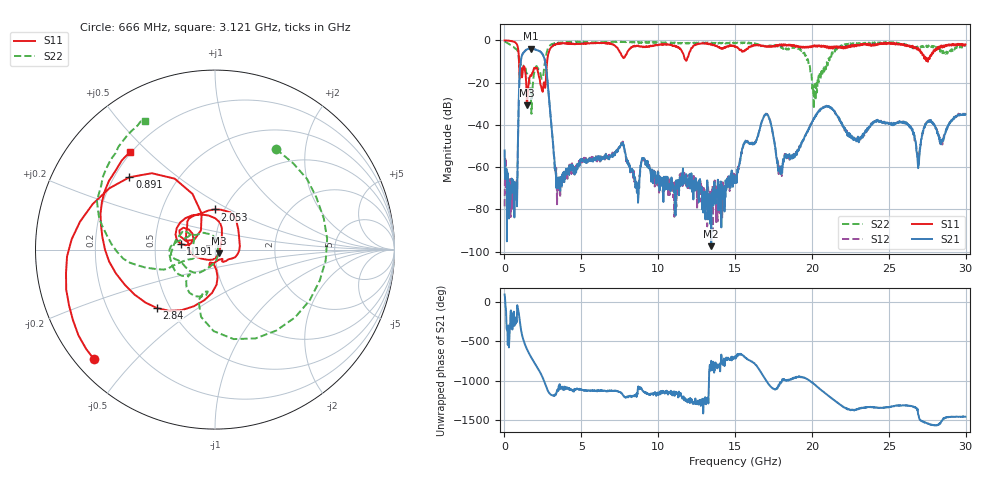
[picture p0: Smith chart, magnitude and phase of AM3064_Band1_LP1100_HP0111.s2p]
# Hz S DB R 50.0
!freq dBS11 angS11 dBS21 angS21 dBS12 angS12 dBS22 angS22
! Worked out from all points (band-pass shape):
!   1600 points, 10 MHz to 29.98 GHz, reference 50 ohm
!   highest |S21| = -3.83 dB at 1.697 GHz (marker M1); lowest = -97.4 dB at 13.45 GHz (marker M2)
!   |S21| within 3 dB of the highest: 1.157 GHz to 2.5 GHz (1.344 GHz wide, 73.5 % of centre)
!   lowest |S11| = -30.7 dB at 1.472 GHz (marker M3), VSWR 1.06, Z = 52.1 - j2.12 ohm
!   |S11| at or under -10 dB: 949.5 MHz to 2.776 GHz (1.827 GHz wide, 98.1 % of centre); 27.5335 GHz to 27.54578 GHz (12.27 MHz wide, 0.0446 % of centre)
!   |S22| runs from -34.8 to -0.5 dB; largest |S21 - S12| = 0.01
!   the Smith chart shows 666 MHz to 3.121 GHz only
!   S11 on the Smith chart (normalised r, x): 666 MHz: 0.05, -0.38; 891 MHz: 0.26, +0.34; 1.191 GHz: 0.68, +0.04; 2.053 GHz: 0.90, +0.43; 2.84 GHz: 0.42, -0.35; 3.121 GHz: 0.19, +0.44
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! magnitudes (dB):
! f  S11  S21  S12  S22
! 10 MHz  0.0  -52.1  -78.5  -0.5
! 666 MHz  -0.8  -75.4  -72.5  -3.7
! 891 MHz  -4.1  -42.7  -42.5  -5.9
! 1.191 GHz  -14.3  -6.3  -6.2  -13.1
! 1.472 GHz  -30.7  -4.2  -4.2  -15.8
! 1.697 GHz  -16.5  -3.8  -3.9  -23.7
! 2.053 GHz  -13.0  -4.5  -4.4  -12.4
! 2.84 GHz  -6.8  -22.5  -22.4  -3.5
! 3.121 GHz  -2.8  -45.7  -45.9  -1.8
! 3.534 GHz  -1.6  -65.6  -65.3  -1.1
! 5.015 GHz  -1.5  -56.1  -57.9  -0.7
! 7.639 GHz  -7.3  -48.4  -48.7  -0.7
! 8.613 GHz  -2.6  -71.9  -68.8  -0.9
! 10 GHz  -2.1  -62.3  -64.3  -1.0
! 13.45 GHz  -1.8  -97.4  -80.5  -1.2
! 15 GHz  -2.9  -64.8  -63.7  -1.4
! 16.97 GHz  -2.8  -35.1  -35.0  -2.7
! 17.95 GHz  -2.3  -62.4  -60.9  -2.8
! 19.99 GHz  -3.2  -38.9  -38.9  -18.0
! 25 GHz  -1.1  -39.2  -39.4  -1.1
! 26.93 GHz  -3.9  -59.2  -59.1  -3.7
! 29.98 GHz  -1.9  -35.0  -35.0  -2.9
